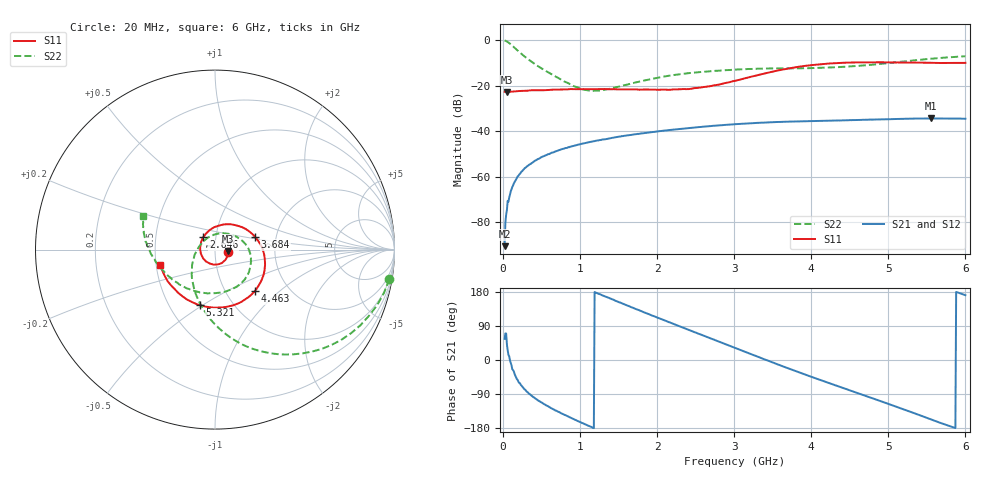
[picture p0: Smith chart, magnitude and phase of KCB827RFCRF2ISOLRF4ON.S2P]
!Agilent Technologies,E5071B,JP1KK00126,A.08.11
!Date: Tue May 06 07:28:38 2014
!Data & Calibration Information:
!Freq	S11:SOLT2(ON)	S21:SOLT2(ON)	S12:SOLT2(ON)	S22:SOLT2(ON)
# Hz S dB R 50
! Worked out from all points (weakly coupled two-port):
!   600 points, 20 MHz to 6 GHz, reference 50 ohm
!   highest |S21| = -34.40 dB at 5.551 GHz (marker M1); lowest = -90.6 dB at 20 MHz (marker M2)
!   lowest |S11| = -22.8 dB at 49.95 MHz (marker M3), VSWR 1.16, Z = 57.8 - j0.913 ohm
!   |S11| at or under -10 dB: start of sweep to 4.393 GHz; 5.647 GHz to 5.785 GHz (137.2 MHz wide, 2.4 % of centre); 5.865 GHz to 5.984 GHz (118.9 MHz wide, 2.01 % of centre)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
!   |S22| runs from -22.4 to -0.1 dB; largest |S21 - S12| = 0.00016
!   S11 on the Smith chart (normalised r, x): 20 MHz: 1.15, -0.03; 2.646 GHz: 0.87, +0.12; 3.684 GHz: 1.55, +0.23; 4.463 GHz: 1.36, -0.70; 5.321 GHz: 0.71, -0.49; 6 GHz: 0.53, -0.10
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2e7  -22.70 -11.5  -90.64 55.7  -85.34 74.2  -0.13 -9.6
4.994992e7  -22.79 -6.2  -74.69 41.0  -75.37 50.8  -0.60 -23.3
8.988314e7  -22.71 -6.9  -67.94 -1.3  -68.61 -0.1  -1.54 -39.4
1.397997e8  -22.57 -9.2  -63.03 -30.1  -62.92 -35.2  -3.03 -56.0
2.196661e8  -22.35 -13.5  -58.77 -61.4  -58.71 -62.1  -5.49 -76.0
3.294825e8  -22.20 -22.0  -55.06 -87.2  -55.01 -87.8  -8.51 -95.7
4.293155e8  -22.04 -27.6  -52.82 -102.9  -52.82 -102.9  -10.91 -110.4
5.690818e8  -21.96 -39.0  -50.45 -120.6  -50.50 -120.7  -13.82 -129.1
1.018331e9  -21.53 -72.8  -45.65 -165.6  -45.66 -165.2  -21.56 159.7
1.267913e9  -21.53 -93.5  -43.92 172.6  -43.90 172.3  -22.18 107.9
2.016661e9  -21.83 -157.7  -40.11 110.9  -40.08 110.6  -16.47 23.8
2.40601e9  -21.54 161.8  -38.69 79.8  -38.67 79.9  -14.54 0.7
2.645609e9  -20.46 133.4  -37.92 60.7  -37.92 60.6  -13.80 -12.3
3.014992e9  -17.86 88.1  -37.00 31.5  -36.99 31.4  -12.96 -32.1
3.344441e9  -15.07 50.9  -36.31 5.6  -36.34 5.4  -12.54 -48.8
3.683873e9  -12.62 17.5  -35.89 -20.8  -35.88 -21.0  -12.37 -68.0
4.013322e9  -10.95 -11.5  -35.61 -45.3  -35.61 -45.5  -12.30 -89.6
4.462571e9  -9.88 -46.2  -35.25 -77.4  -35.23 -77.4  -11.66 -121.3
5.011653e9  -9.78 -83.5  -34.78 -116.5  -34.78 -116.8  -10.04 -158.9
5.321135e9  -9.89 -105.1  -34.51 -139.3  -34.51 -139.6  -8.92 -176.3
5.550751e9  -9.97 -123.0  -34.40 -156.5  -34.40 -156.6  -8.17 172.9
6e9  -9.97 -164.3  -34.58 171.0  -34.54 171.0  -7.10 154.5
